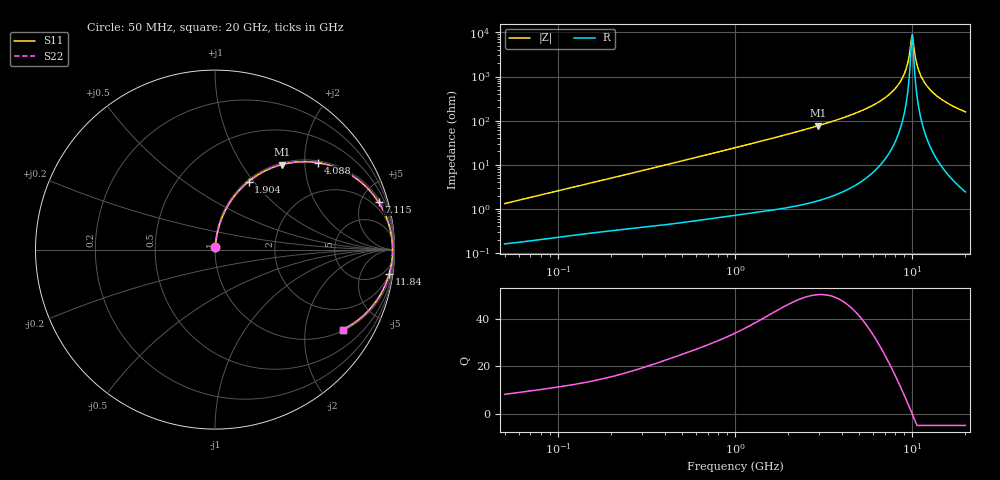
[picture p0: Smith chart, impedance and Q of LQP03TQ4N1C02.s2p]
!Murata Part Number: LQP03TQ4N1C02
!These Parameters are Measured in Series Mode Connection
!  o--[Z]--o
!Port1  Port2
!  o-------o
!Freq. Start=50[MHz] Stop=20[GHz], 401[Steps]
# Hz S RI R 50
!Freq.(Hz) S11(Real) S11(Imag) S21(Real) S21(Imag) S12(Real) S12(Imag) S22(Real) S22(Imag)
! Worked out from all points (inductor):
!   401 points, 50 MHz to 20 GHz, reference 50 ohm
!   read as one part in series: L = 4.12 nH near 51.52 MHz
!   highest Q = 50.3 at 2.94 GHz (marker M1), where L = 4.14 nH
!   self-resonance near 9.892 GHz
!   S11 on the Smith chart (normalised r, x): 50 MHz: 1.00, +0.03; 1.904 GHz: 1.02, +0.94; 4.088 GHz: 1.05, +2.33; 7.115 GHz: 1.28, +6.81; 11.84 GHz: 2, -14; 20 GHz: 1.05, -3.17
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5e7  0.00177 0.013  0.9982 -0.013  0.9982 -0.013  0.00177 0.013
1.364002e8  0.00381 0.034  0.9962 -0.034  0.9962 -0.034  0.00381 0.034
3.721004e8  0.0123 0.0894  0.9877 -0.0894  0.9877 -0.0894  0.0123 0.0894
1e9  0.0614 0.2258  0.9386 -0.2258  0.9386 -0.2258  0.0614 0.2258
1.904239e9  0.1867 0.3788  0.8133 -0.3788  0.8133 -0.3788  0.1867 0.3788
2.728004e9  0.3323 0.4612  0.6677 -0.4612  0.6677 -0.4612  0.3323 0.4612
2.940159e9  0.3714 0.4734  0.6286 -0.4734  0.6286 -0.4734  0.3714 0.4734
4.087748e9  0.5741 0.484  0.4259 -0.484  0.4259 -0.484  0.5741 0.484
5.598765e9  0.7827 0.3991  0.2173 -0.3991  0.2173 -0.3991  0.7827 0.3991
7.114996e9  0.9116 0.2638  0.0884 -0.2638  0.0884 -0.2638  0.9116 0.2638
7.442007e9  0.93 0.2327  0.07 -0.2327  0.07 -0.2327  0.93 0.2327
8.264682e9  0.9639 0.1546  0.0361 -0.1546  0.0361 -0.1546  0.9639 0.1546
8.907419e9  0.9797 0.0953  0.0203 -0.0953  0.0203 -0.0953  0.9797 0.0953
9.316812e9  0.9856 0.0588  0.0144 -0.0588  0.0144 -0.0588  0.9856 0.0588
9.745021e9  0.9888 0.0219  0.0112 -0.0219  0.0112 -0.0219  0.9888 0.0219
1.004137e10  0.9893 -0.00276  0.0107 0.00276  0.0107 0.00276  0.9893 -0.00276
1.019291e10  0.9892 -0.0151  0.0108 0.0151  0.0108 0.0151  0.9892 -0.0151
1.082228e10  0.9854 -0.0643  0.0146 0.0643  0.0146 0.0643  0.9854 -0.0643
1.183995e10  0.9705 -0.1367  0.0295 0.1367  0.0295 0.1367  0.9705 -0.1367
1.295331e10  0.9452 -0.2056  0.0548 0.2056  0.0548 0.2056  0.9452 -0.2056
1.460232e10  0.8967 -0.2894  0.1033 0.2894  0.1033 0.2894  0.8967 -0.2894
2e10  0.7122 -0.4452  0.2878 0.4452  0.2878 0.4452  0.7122 -0.4452
